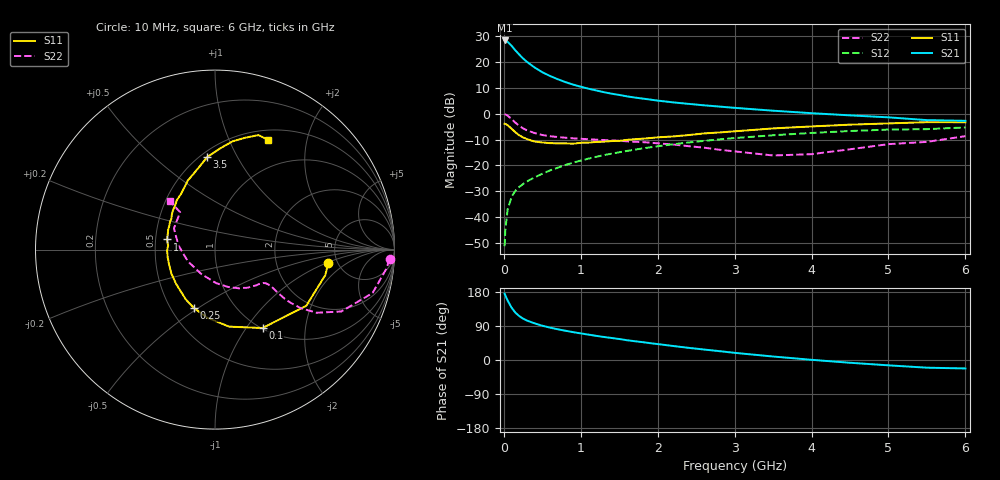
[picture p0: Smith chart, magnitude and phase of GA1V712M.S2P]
! Infineon Technologies  Discrete & RF Semiconductors
! BF775
! Si NPN RF Bipolar Junction Transistor in SOT23
! VCE = 1.75 V  IC = 12 mA
! Common Emitter S-Parameters:  May  1996
# GHz  S  MA  R  50
!  f  S11  S21  S12  S22
! GHz  MAG  ANG  MAG  ANG  MAG  ANG  MAG  ANG
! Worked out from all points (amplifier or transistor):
!   36 points, 10 MHz to 6 GHz, reference 50 ohm
!   highest |S21| = 28.1 dB at 10 MHz (marker M1)
!   |S21| within 3 dB of that: start of sweep to 126.7 MHz
!   unconditionally stable (mu >= 1): 468.1 MHz to 3.959 GHz; 5.483 GHz to 5.537 GHz
!   at 250 MHz: K = 0.77, MSG = 24.2 dB, |S12| = -27.2 dB
!   at 1.4 GHz: K = 1.13, MAG = 9.3 dB, |S12| = -15.5 dB
!   at 6 GHz: K = 0.99, MSG = 1.3 dB, |S12| = -5.3 dB
!   S11 on the Smith chart (normalised r, x): 10 MHz: 4.19, -1.07; 100 MHz: 1.01, -1.19; 250 MHz: 0.65, -0.48; 1 GHz: 0.57, +0.07; 3.5 GHz: 0.54, +0.76; 6 GHz: 0.62, +1.41
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0.01  0.6353 -6.9  25.51 175.1  0.0028 88.0  0.9739 -3.1
0.02  0.6309 -13.0  25.1 170.1  0.006 78.4  0.9606 -6.4
0.05  0.5971 -31.6  23.91 156.6  0.0144 76.2  0.9107 -15.4
0.1  0.511 -58.8  20.14 138.4  0.0248 67.5  0.7837 -26.1
0.15  0.4361 -79.7  16.41 125.0  0.0327 62.9  0.6676 -31.8
0.2  0.3815 -96.6  13.68 116.0  0.0386 61.4  0.5805 -34.3
0.25  0.3471 -109.4  11.48 109.1  0.0439 60.9  0.5176 -35.1
0.3  0.3222 -120.2  9.881 104.1  0.0493 61.5  0.4762 -35.2
0.4  0.289 -138.6  7.699 96.7  0.0591 63.1  0.421 -34.4
0.5  0.2775 -151.1  6.246 90.4  0.0693 63.9  0.3861 -33.5
0.6  0.2693 -161.4  5.282 85.5  0.0803 64.5  0.3665 -33.1
0.7  0.2671 -170.5  4.582 81.1  0.0907 64.8  0.3533 -33.2
0.8  0.2672 -179.1  4.028 77.2  0.1022 64.5  0.3422 -33.5
1  0.2735 168.0  3.282 70.2  0.1244 64.1  0.3268 -34.8
1.1  0.2759 163.1  3.012 67.0  0.1356 63.4  0.3203 -36.4
1.3  0.2873 152.5  2.578 60.8  0.1582 61.8  0.3089 -38.9
1.6  0.3113 140.4  2.141 52.2  0.1907 58.8  0.2917 -44.3
2.2  0.3623 121.7  1.641 37.0  0.256 52.0  0.2536 -58.3
3.5  0.5173 94.8  1.134 9.2  0.3821 34.7  0.1559 -119.5
4.5  0.6109 80.8  0.922 -7.3  0.461 21.0  0.2051 173.4
5.5  0.6824 69.2  0.747 -20.3  0.5009 6.7  0.2847 133.0
6  0.6797 64.1  0.724 -22.3  0.5406 2.7  0.3671 132.9
